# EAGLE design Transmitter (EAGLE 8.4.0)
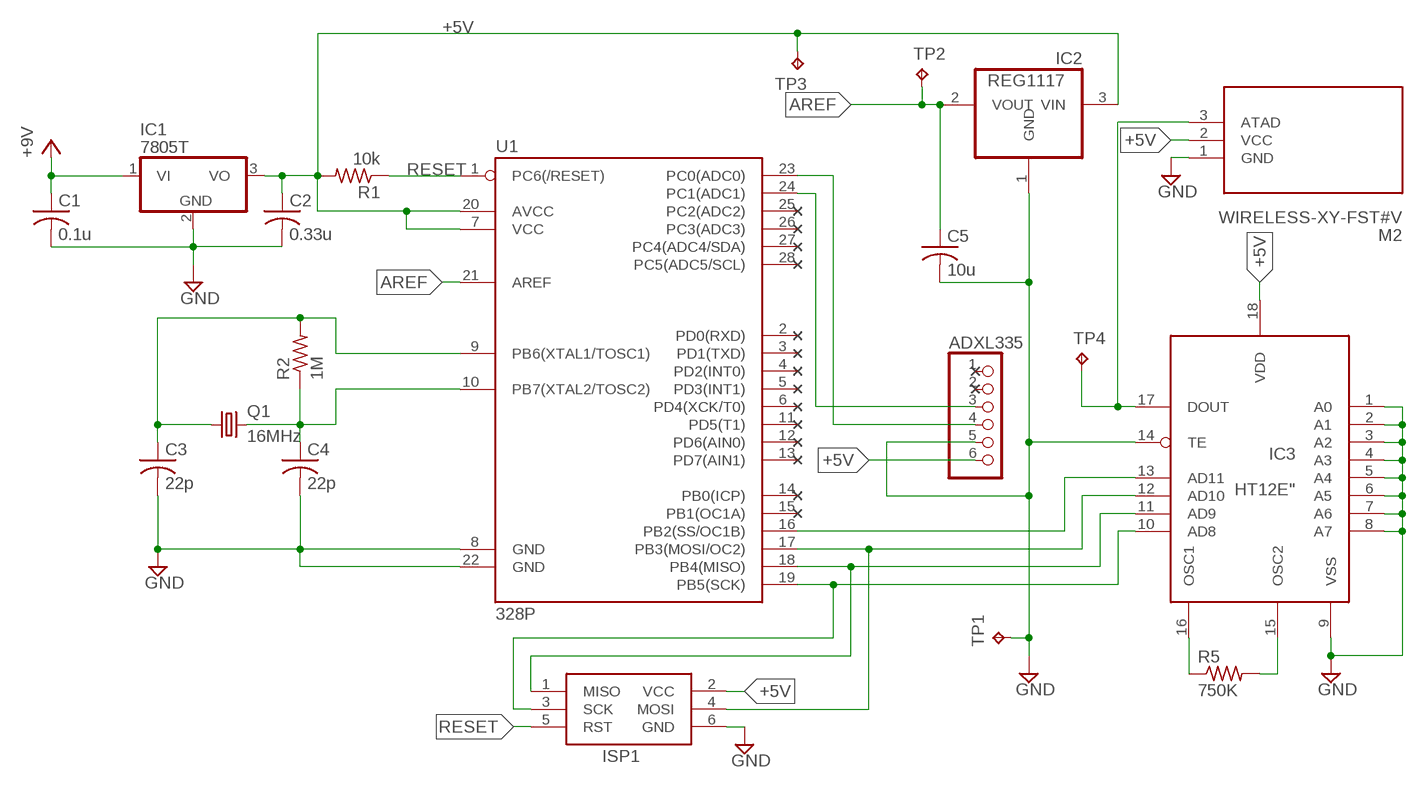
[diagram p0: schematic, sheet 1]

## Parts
ADXL335  PINHD-1X6  [1X06]
C1  0.1u  C-USC0805  [C0805]
C2  0.33u  C-USC0805  [C0805]
C3  22p  C-USC0805  [C0805]
C4  22p  C-USC0805  [C0805]
C5  10u  C-USC0805  [C0805]
IC1  7805T  [TO220H]
IC2  REG1117  [SOT223]
IC3  HT12E"  [18-DIP-A]
ISP1  AVRISP-6  [AVRISP]
M2  WIRELESS-XY-FST#V  [WIRELESS-XY-FST#V]
Q1  16MHz  CRYTALHC49S  [HC49/S]
R1  10k  R-US_R0805  [R0805]
R2  1M  R-US_R0805  [R0805]
R5  750K  R-US_R0805  [R0805]
TP1  TPB1,27  [B1,27]
TP2  TPB1,27  [B1,27]
TP3  TPB1,27  [B1,27]
TP4  TPB1,27  [B1,27]
U1  328P  ATMEGA328P_PDIP  [DIP28]

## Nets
+5V: ADXL335.6 C2.1 IC1.3(VO) IC2.3(VIN) IC3.18(VDD) ISP1.2(VCC) M2.2(VCC) R1.2 TP3.TP U1.7(VCC) U1.20(AVCC)
AD08: IC3.10(AD8) ISP1.3(SCK) U1.19(PB5(SCK))
AREF: C5.1 IC2.2(VOUT) TP2.TP U1.21(AREF)
GND: ADXL335.5 C1.2 C2.2 C3.2 C4.2 C5.2 IC1.2(GND) IC2.1(GND) IC3.1(A0) IC3.2(A1) IC3.3(A2) IC3.4(A3) IC3.5(A4) IC3.6(A5) IC3.7(A6) IC3.8(A7) IC3.9(VSS) IC3.14(TE) ISP1.6(GND) M2.1(GND) TP1.TP U1.8(GND) U1.22(GND)
N$1: C3.1 Q1.1 R2.2 U1.9(PB6(XTAL1/TOSC1))
N$2: IC3.11(AD9) ISP1.1(MISO) U1.18(PB4(MISO))
N$4: C4.1 Q1.2 R2.1 U1.10(PB7(XTAL2/TOSC2))
N$5: IC3.16(OSC1) R5.1
N$6: IC3.15(OSC2) R5.2
N$8: IC3.13(AD11) U1.16(PB2(SS/OC1B))
N$9: IC3.12(AD10) ISP1.4(MOSI) U1.17(PB3(MOSI/OC2))
N$11: ADXL335.3 U1.24(PC1(ADC1))
N$12: ADXL335.4 U1.23(PC0(ADC0))
N$13: IC3.17(DOUT) M2.3(ATAD) TP4.TP
RESET: ISP1.5(RST) R1.1 U1.1(PC6(/RESET))
VCC: C1.1 IC1.1(VI) ; supply symbol labelled +9V
Unconnected: ADXL335.1 ADXL335.2 U1.2(PD0(RXD)) U1.3(PD1(TXD)) U1.4(PD2(INT0)) U1.5(PD3(INT1)) U1.6(PD4(XCK/T0)) U1.11(PD5(T1)) U1.12(PD6(AIN0)) U1.13(PD7(AIN1)) U1.14(PB0(ICP)) U1.15(PB1(OC1A)) U1.25(PC2(ADC2)) U1.26(PC3(ADC3)) U1.27(PC4(ADC4/SDA)) U1.28(PC5(ADC5/SCL))

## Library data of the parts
ADXL335 = adafruit:PINHD-1X6: PIN HEADER
C1-C5 = adafruit:C-US: CAPACITOR, American symbol
IC1 = linear:78*: Positive VOLTAGE REGULATOR Source: http://cache.national.com/ds/LM/LM78L05.pdf http://www.fairchildsemi.com/ds/LM/LM7805.pdf
IC2 = burr-brown:REG1117: 800mA and 1A Low Dropout (LDO) Positive Regulator 1.8V, 2.5V, 2.85V, 3.3V, 5V, and Adj; MPN: REG1117; OC_FARNELL: 1097566; OC_NEWARK: 14P6981
IC3 = holtek:HT12E: transmitter = encoder ic
ISP1 = adafruit:AVRISP: AVR ISP HEADER Standard 6 pin header for AVR programming
M2 = diy-modules:WIRELESS-XY-FST#V: RF Wireless XY-FST Transmitter vertically mounted Click here to find device on ebay.com Note: Sold together with receiver.
Q1 = crystal:CRYTAL: CRYSTAL
R1 R2 R5 = adafruit:R-US_: RESISTOR, American symbol
TP1-TP4 = testpad:TP: Test pad
U1 = SparkFun-IC-Microcontroller:ATMEGA328P_PDIP: Atmel 328P Through hole ATMEGA328P uC used in the Arduino 32kb flash, 1k EEPROM, 2k SRAM Datasheet SparkFun Products Storefront component: AVR 28 Pin 20MHz 32K 6A/D - ATMega328P (COM-09061) SparkFun Simon Says - Through-Hole Soldering Kit (KIT-10547) SparkFun Learn to Solder - Simon Says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; PROD_ID: IC-09136

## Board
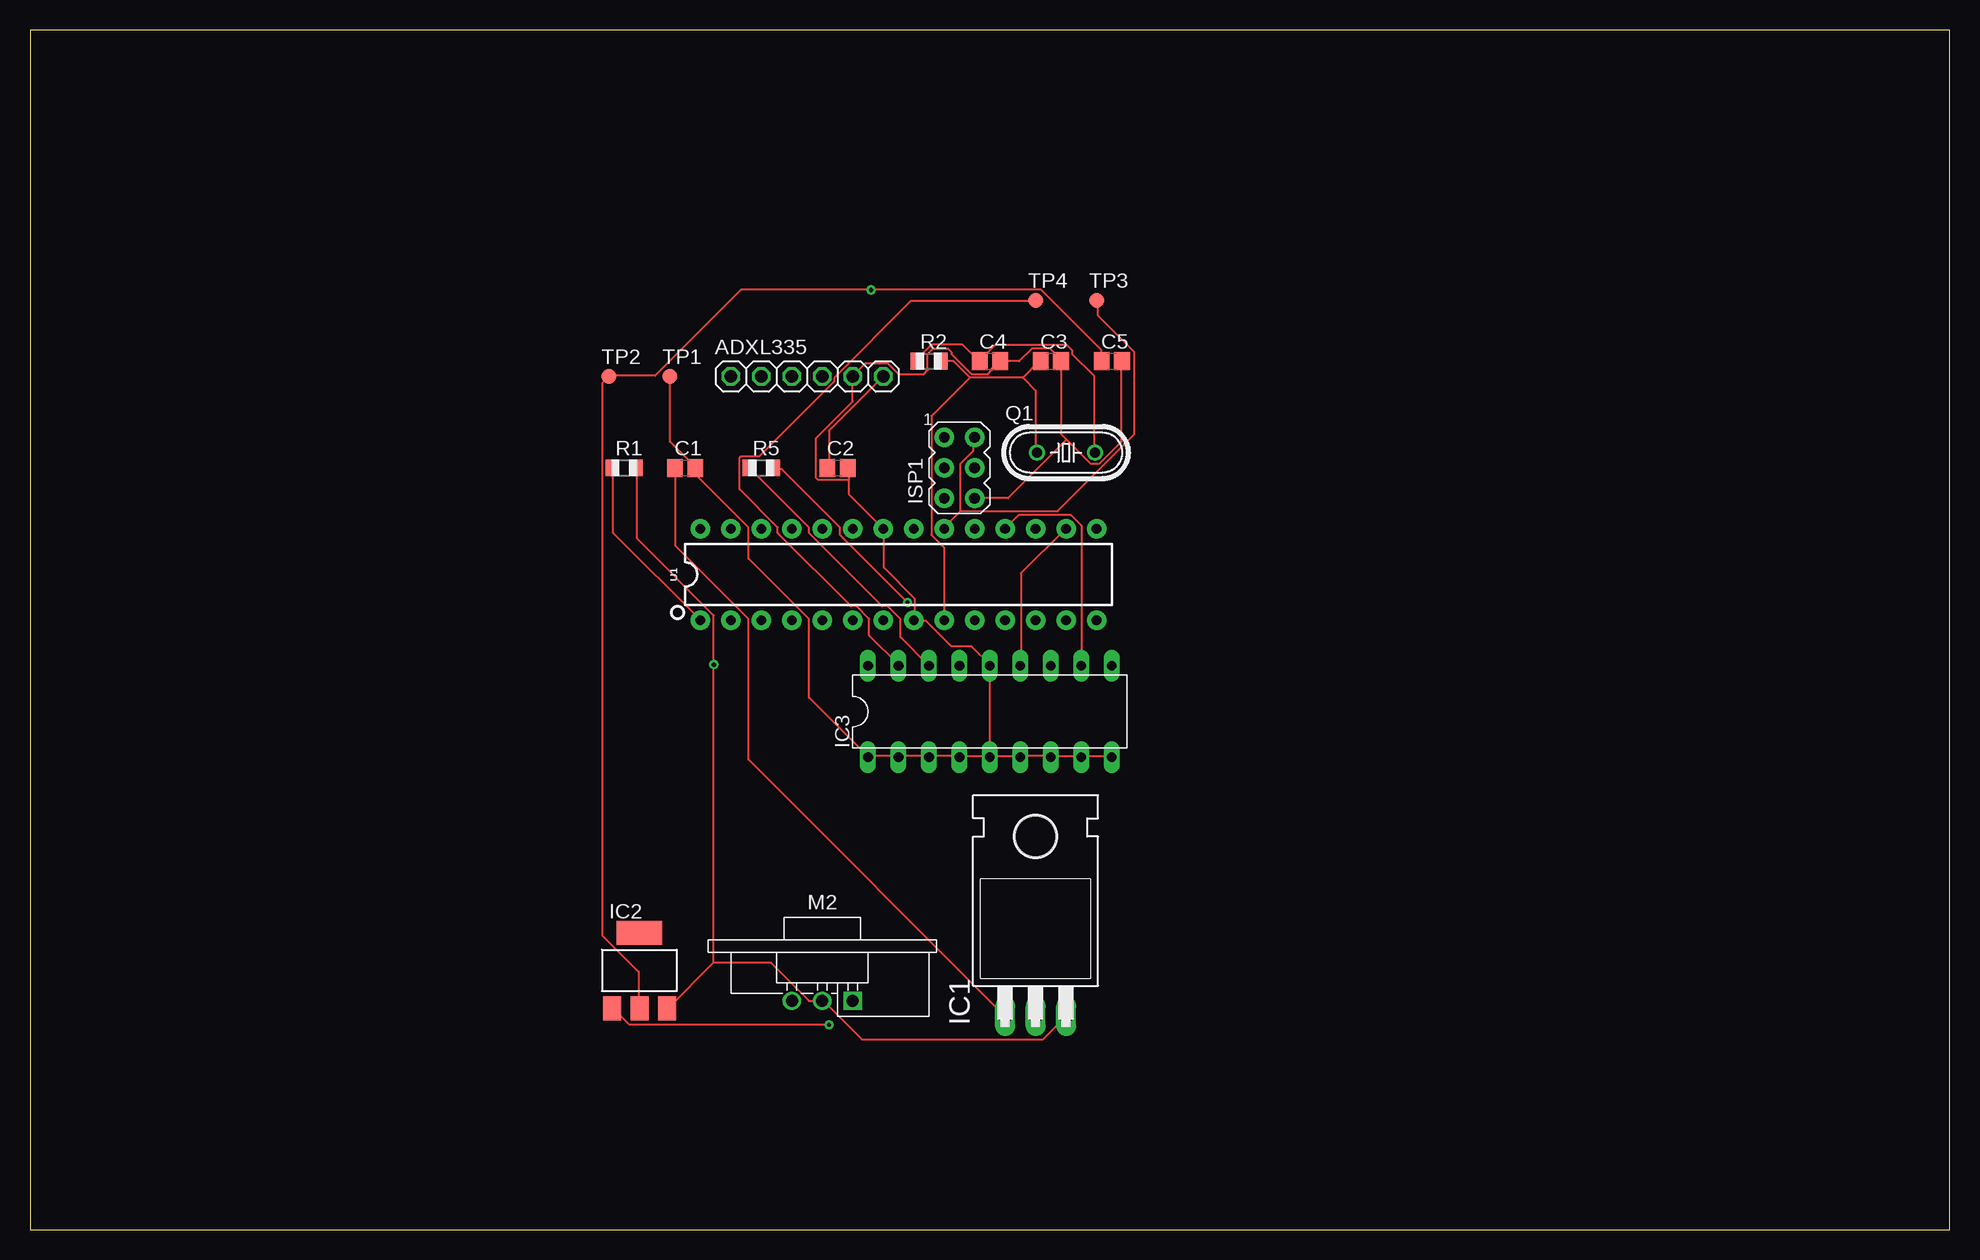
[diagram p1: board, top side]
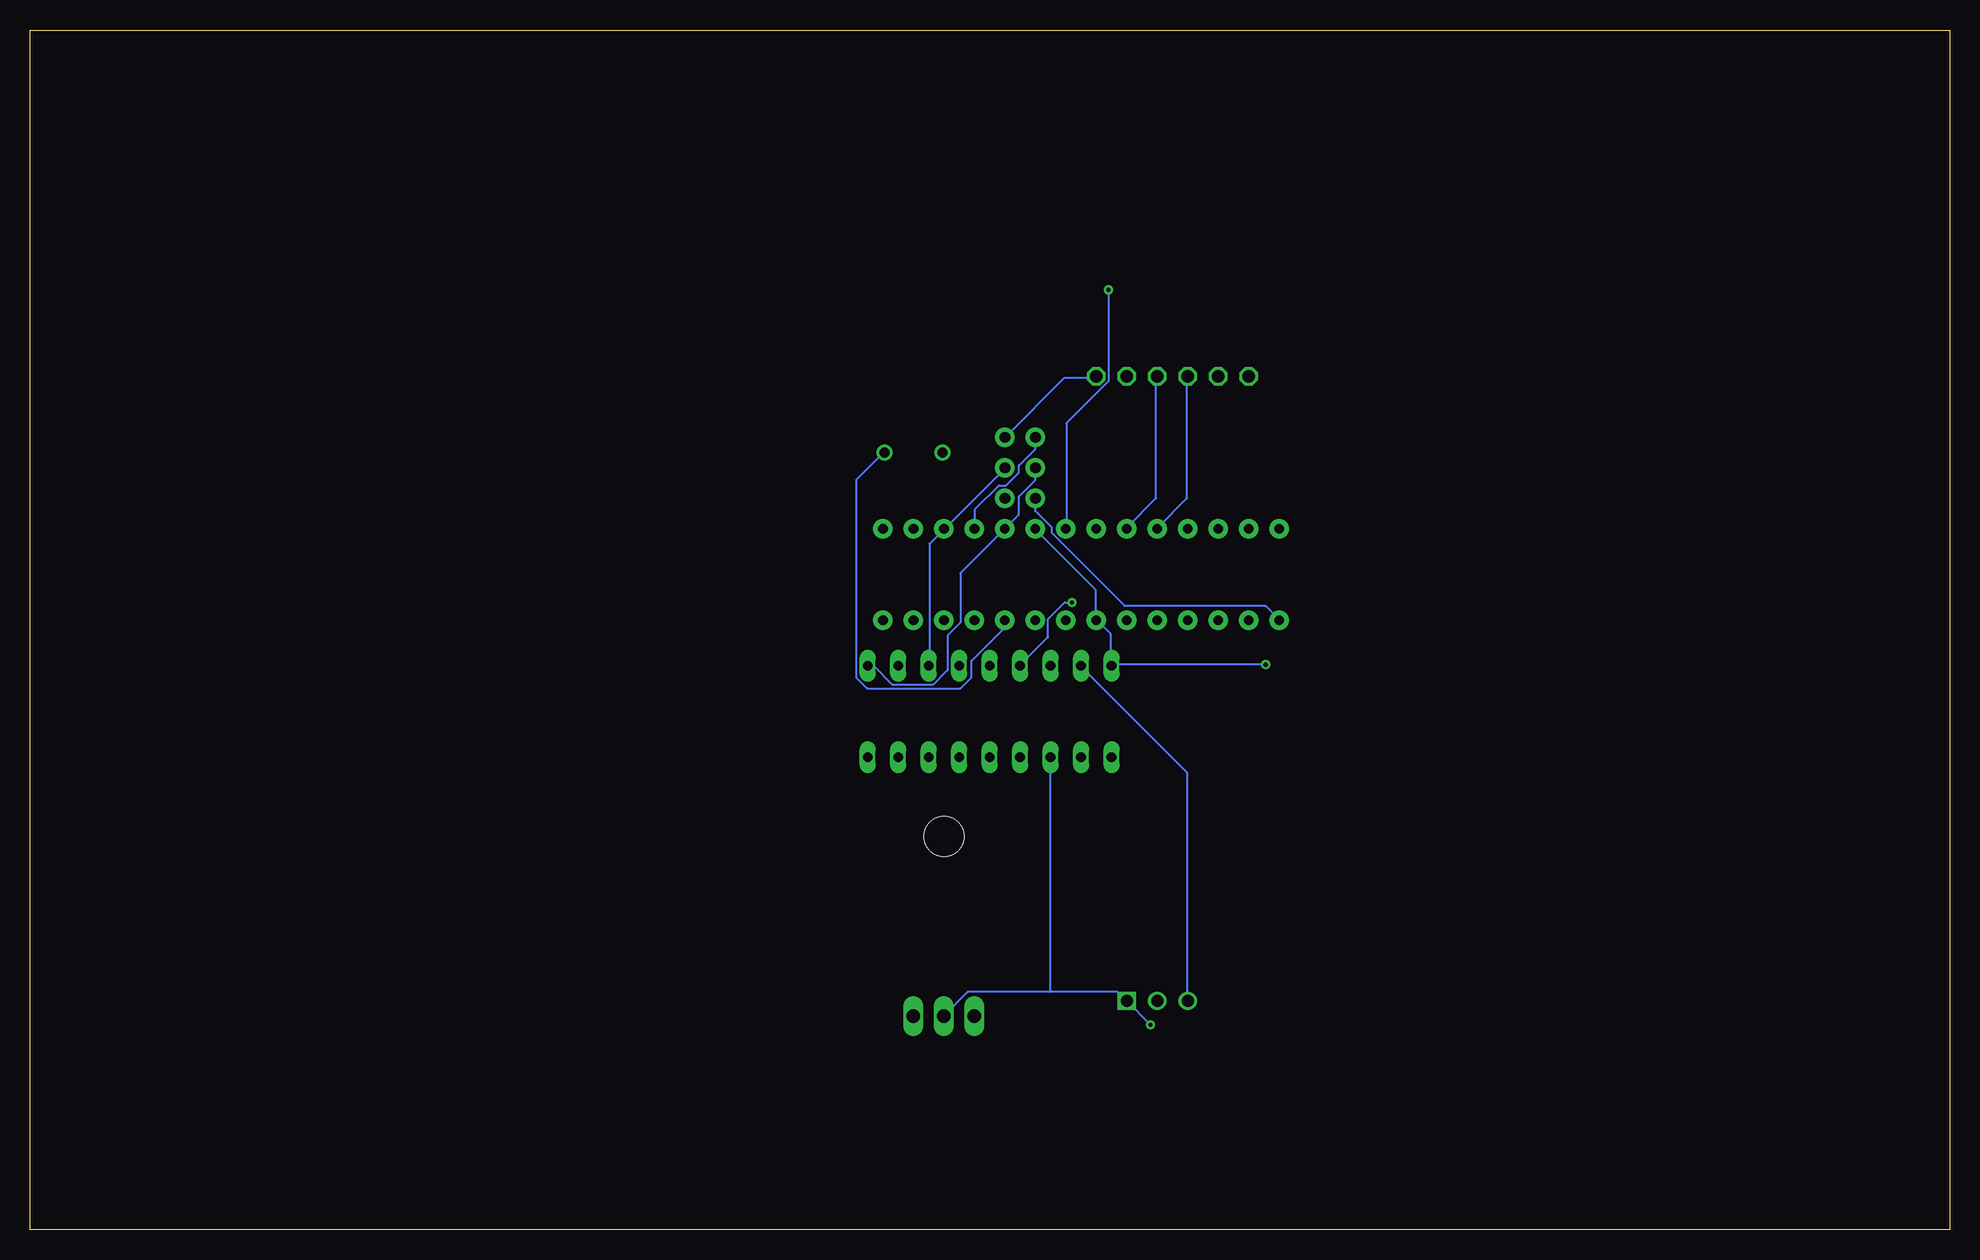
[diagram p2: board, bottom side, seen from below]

Size 160 x 100 mm. Coordinates in mm from the lower left corner, seen from the top.
Outline: 0,0 160,0 160,100 0,100 0,0
Copper layers (1*16): Top 0.035mm / dielectric 1.5mm / Bottom 0.035mm
Design rules "default": minimum track width 6mil, minimum drill 0.35mm, track to track 6mil, track to pad 6mil, pad to pad 6mil, via to via 6mil, smd to smd 6mil, copper to edge 40mil, drill to drill 6mil, minimum pad ring 10mil, minimum via ring 8mil, stop-mask expansion 4mil, vias tented up to drill 0mil, thermal gap 10mil

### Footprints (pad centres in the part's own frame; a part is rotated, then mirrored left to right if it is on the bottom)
1X06 = drill 1.016 octagon: 1 -6.35,0; 2 -3.81,0; 3 -1.27,0; 4 1.27,0; 5 3.81,0; 6 6.35,0
C0805 = smd 1.3 x 1.5: 1 -0.85,0; 2 0.85,0
TO220H = drill 1.118 long: 1 -2.54,-10.16; 2 0,-10.16; 3 2.54,-10.16 | hole 3.302: 0,4.826
SOT223 = smd 1.499 x 2.007: 1 -2.261,-3.15; 2 0.025,-3.15; 3 2.311,-3.15 | smd 3.81 x 2.007: 4 0,3.15
18-DIP-A = drill 0.813 long: 1 -10.16,-3.81; 2 -7.62,-3.81; 3 -5.08,-3.81; 4 -2.54,-3.81; 5 0,-3.81; 6 2.54,-3.81; 7 5.08,-3.81; 8 7.62,-3.81; 9 10.16,-3.81; 10 10.16,3.81; 11 7.62,3.81; 12 5.08,3.81; 13 2.54,3.81; 14 0,3.81; 15 -2.54,3.81; 16 -5.08,3.81; 17 -7.62,3.81; 18 -10.16,3.81
AVRISP = drill 0.9 pad 1.626: 1 -1.27,2.54; 2 1.27,2.54; 3 -1.27,0; 4 1.27,0; 5 -1.27,-2.54; 6 1.27,-2.54
WIRELESS-XY-FST#V = drill 1 square: 1 2.54,0 | drill 1: 2 0,0; 3 -2.54,0
HC49/S = drill 0.813: 1 -2.413,0; 2 2.413,0
R0805 = smd 1.1 x 1.4: 1 -1,0; 2 1,0
B1,27 = smd 1.27 x 1.27: TP 0,0
DIP28 = drill 0.813 pad 1.626: 1 -16.51,-3.81; 2 -13.97,-3.81; 3 -11.43,-3.81; 4 -8.89,-3.81; 5 -6.35,-3.81; 6 -3.81,-3.81; 7 -1.27,-3.81; 8 1.27,-3.81; 9 3.81,-3.81; 10 6.35,-3.81; 11 8.89,-3.81; 12 11.43,-3.81; 13 13.97,-3.81; 14 16.51,-3.81; 15 16.51,3.81; 16 13.97,3.81; 17 11.43,3.81; 18 8.89,3.81; 19 6.35,3.81; 20 3.81,3.81; 21 1.27,3.81; 22 -1.27,3.81; 23 -3.81,3.81; 24 -6.35,3.81; 25 -8.89,3.81; 26 -11.43,3.81; 27 -13.97,3.81; 28 -16.51,3.81

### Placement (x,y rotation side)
ADXL335  64.77,71.12 0 top
C1  54.61,63.5 0 top
C2  67.31,63.5 0 top
C3  85.09,72.39 0 top
C4  80.01,72.39 0 top
C5  90.17,72.39 0 top
IC1  83.82,27.94 0 top
IC2  50.8,21.59 0 top
IC3  80.01,43.18 0 top
ISP1  77.47,63.5 0 top
M2  66.04,19.05 0 top
Q1  86.36,64.77 0 top
R1  49.53,63.5 0 top
R2  74.93,72.39 0 top
R5  60.96,63.5 0 top
TP1  53.34,71.12 0 top
TP2  48.26,71.12 0 top
TP3  88.9,77.47 0 top
TP4  83.82,77.47 0 top
U1  72.39,54.61 0 top

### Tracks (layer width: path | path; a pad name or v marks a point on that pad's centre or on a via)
+5V  (via drill 0.35)
  Top 0.152: ADXL335.6 66.6,66.6 66.6,63.55 C2.1 | 77.57,59.89 85.65,59.89 92.05,66.29 92.05,73.15 89,76.2 89,77.42 TP3.TP | 77.57,59.89 76.2,58.52 U1.20 | 77.57,59.89 77.57,63.86 78.64,64.92 78.64,65.99 ISP1.2 | 57,22.25 v57,47.09 57,51.21 50.6,57.61 50.6,63.4 R1.2 | 57,22.25 53.19,18.44 IC2.3 | 57,22.25 61.72,22.25 64.92,19.05 M2.2 66.14,19.05 69.34,15.85 84.43,15.85 IC1.3
  Bottom 0.152: U1.20 76.2,58.37 71.17,53.34 71.17,50.9 U1.7 71.02,50.75 69.95,49.68 69.95,47.09 IC3.18 69.8,47.09 v57,47.09 | ISP1.2 73.76,71.02 71.17,71.02 ADXL335.6
AD08
  Bottom 0.152: IC3.10 90.07,46.94 89.61,46.94 88.09,45.41 84.73,45.41 83.52,46.63 83.52,49.53 82.45,50.6 82.45,54.71 U1.19 77.57,59.59 77.57,61.11 76.2,62.48 ISP1.3
AREF  (via drill 0.35)
  Top 0.152: C5.1 89.31,72.39 89.31,73.3 84.28,78.33 v70.1,78.33 59.28,78.33 52.12,71.17 48.31,71.17 TP2.TP 47.7,70.56 47.7,24.54 50.75,21.49 50.75,18.44 IC2.2
  Bottom 0.152: v70.1,78.33 70.1,70.71 73.61,67.21 73.61,58.52 U1.21
GND  (via drill 0.35)
  Top 0.152: v66.6,17.07 49.99,17.07 48.62,18.44 IC2.1 | 86.41,65.84 85.95,66.29 85.95,72.39 C3.2 85.8,72.39 85.8,72.69 85.04,73.46 83.52,73.46 82.45,72.39 C4.2 80.77,72.39 80.16,71.78 80.16,71.63 79.86,71.32 78.49,71.32 76.81,73 76.81,73.15 76.5,73.46 75.29,73.46 74.83,73 74.83,71.63 74.52,71.32 72.39,71.32 71.48,72.24 69.65,72.24 68.58,71.17 ADXL335.5 68.58,69.04 65.53,65.99 65.53,62.64 65.68,62.48 68.28,62.48 | 86.41,65.84 88.39,63.86 89.15,63.86 90.98,65.68 90.98,72.39 C5.2 | ISP1.6 81.53,60.96 86.41,65.84 | 68.28,62.48 68.28,61.27 U1.22 71.17,58.37 71.17,55.17 73.76,52.58 73.76,50.9 U1.8 73.76,50.75 74.68,50.75 76.81,48.62 78.49,48.62 80.01,47.09 IC3.14 80.01,39.47 | 68.28,62.48 68.28,63.4 C2.2 | 87.63,39.47 85.19,39.47 IC3.7 85.04,39.47 82.6,39.47 IC3.6 82.45,39.47 80.01,39.47 | 87.63,39.47 90.07,39.47 IC3.9 | 87.63,39.47 IC3.8 | TP1.TP 53.34,65.68 55.47,63.55 C1.2 55.47,63.4 55.47,62.94 59.89,58.52 59.89,55.93 64.92,50.9 64.92,44.35 69.8,39.47 IC3.1 69.95,39.47 72.39,39.47 | 80.01,39.47 77.57,39.47 IC3.4 77.42,39.47 74.98,39.47 IC3.3 74.83,39.47 72.39,39.47 | 72.39,39.47 IC3.2 | 80.01,39.47 IC3.5
  Bottom 0.152: v66.6,17.07 M2.1 69.34,19.81 74.98,19.81 | 74.98,19.81 81.84,19.81 83.82,17.83 IC1.2 | 74.98,19.81 74.98,39.32 IC3.3
N$1
  Top 0.152: R2.2 76.96,72.39 78.33,71.02 | 82.75,71.02 78.33,71.02 | 82.75,71.02 84.12,72.39 C3.1 | 82.75,71.02 83.82,69.95 83.82,64.77 Q1.1 | U1.9 76.2,56.84 75.13,57.91 75.13,67.82 78.33,71.02
N$2
  Top 0.152: IC3.11 87.63,58.67 86.72,59.59 82.45,59.59 U1.18
  Bottom 0.152: ISP1.1 76.2,65.08 77.57,63.7 77.57,63.09 78.64,62.03 79.25,62.03 81.23,60.05 81.23,58.52 U1.18
N$4
  Top 0.152: 79.1,72.39 77.72,73.76 75.13,73.76 74.07,72.69 74.07,72.39 R2.1 | 79.1,72.39 80.47,73.76 86.41,73.76 86.87,73.3 86.87,73 88.7,71.17 88.7,64.77 Q1.2 | 79.1,72.39 C4.1
  Bottom 0.152: U1.10 78.79,50.75 78.79,50.14 81.53,47.4 81.53,46.02 82.45,45.11 90.22,45.11 91.14,46.02 91.14,62.48 88.85,64.77 Q1.2
N$5
  Top 0.152: IC3.16 72.54,49.38 72.54,50.9 71.48,51.97 71.02,51.97 64.92,58.06 64.92,58.52 60.05,63.4 R5.1
N$6  (via drill 0.35)
  Top 0.152: v73.15,52.27 67.51,57.91 67.51,58.52 62.64,63.4 62.03,63.4 R5.2
  Bottom 0.152: v73.15,52.27 73.76,52.27 75.13,50.9 75.13,49.38 77.42,47.09 IC3.15
N$8
  Top 0.152: IC3.13 82.6,47.09 82.6,54.71 86.26,58.37 U1.16
N$9
  Bottom 0.152: 83.82,58.37 85.04,57.15 85.04,47.09 IC3.12 | 83.82,58.37 78.79,63.4 ISP1.4 | 83.82,58.37 U1.17
N$11
  Bottom 0.152: ADXL335.3 63.55,71.02 63.55,60.96 65.99,58.52 U1.24
N$12
  Bottom 0.152: ADXL335.4 66.14,71.02 66.14,60.96 68.58,58.52 U1.23
N$13
  Top 0.152: TP4.TP 83.82,77.42 73.46,77.42 67.06,71.02 67.06,70.71 60.81,64.47 59.28,64.47 59.13,64.31 59.13,61.72 62.33,58.52 62.33,58.06 68.43,51.97 68.89,51.97 69.95,50.9 69.95,49.53 72.39,47.09 IC3.17
  Bottom 0.152: M2.3 63.55,19.05 63.55,38.1 72.39,46.94 IC3.17
RESET
  Top 0.152: U1.1 48.62,58.06 48.62,63.4 R1.1
  Bottom 0.152: ISP1.5 76.2,59.89 74.83,58.52 74.83,58.06 68.73,51.97 57,51.97 55.93,50.9 U1.1
VCC
  Top 0.152: IC1.1 59.89,39.17 59.89,50.9 53.8,57 53.8,63.4 C1.1

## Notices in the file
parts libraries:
SparkFun-IC-Microcontroller: Licensing: Creative Commons ShareAlike 4.0 International - https://creativecommons.org/licenses/by-sa/4.0
diy-modules: Released under the Creative Commons Attribution 4.0 International License: http://creativecommons.org/licenses/by/4.0
